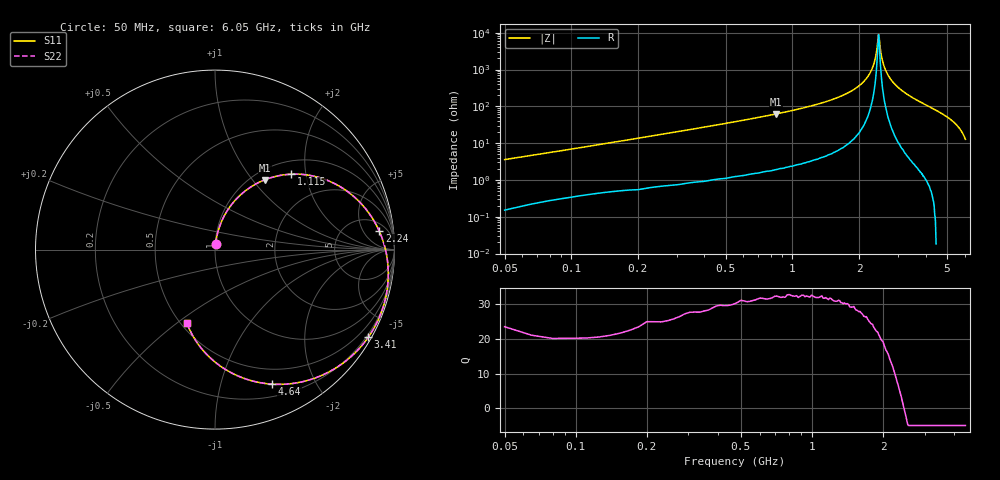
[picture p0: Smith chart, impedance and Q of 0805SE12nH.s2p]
! AVX Thin Film Operation		Date: May 2002
! Description: Accu-L® Series, Thin Film, SMD, RF Inductors
! Part Number: L0805120GEWTR
! 50 MHz  -  6.05 GHz
! Serial Measurements
# mhz S db R 50
!	S11		S21		S12		S22
!	dB	Phase	dB	Phase	dB	Phase	dB	Phase
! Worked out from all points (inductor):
!   401 points, 50 MHz to 6.05 GHz, reference 50 ohm
!   read as 1/Y11, port 2 shorted: L = 10.9 nH near 80 MHz
!   highest Q = 32.5 at 845 MHz (marker M1), where L = 11.7 nH
!   self-resonance near 2.45 GHz
!   S11 on the Smith chart (normalised r, x): 50 MHz: 1.00, +0.07; 1.115 GHz: 1.27, +1.66; 2.24 GHz: 9, +12; 3.41 GHz: 0.12, -3.76; 4.64 GHz: 0.33, -1.46; 6.05 GHz: 0.54, -0.54
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50  -29.56 84.5  -0.01 -2.2  -0.01 -2.2  -29.56 84.5
155  -20.28 80.8  -0.08 -6.4  -0.08 -6.4  -20.28 80.8
305  -14.60 75.2  -0.21 -12.4  -0.21 -12.4  -14.60 75.2
530  -10.07 66.6  -0.54 -21.2  -0.54 -21.2  -10.07 66.6
845  -6.44 54.6  -1.24 -33.1  -1.24 -33.1  -6.44 54.6
1055  -4.84 46.8  -1.88 -40.8  -1.88 -40.8  -4.84 46.8
1115  -4.46 44.6  -2.08 -42.9  -2.09 -42.9  -4.46 44.6
1550  -2.41 29.2  -3.96 -57.9  -3.96 -57.9  -2.41 29.2
2060  -1.03 12.2  -7.26 -74.1  -7.26 -74.1  -1.03 12.2
2240  -0.71 6.4  -8.87 -79.5  -8.87 -79.5  -0.71 6.4
2795  -0.16 -11.0  -17.60 -93.8  -17.60 -93.8  -0.16 -11.0
2960  -0.10 -16.1  -23.82 -93.8  -23.80 -93.8  -0.10 -16.1
3050  -0.09 -18.8  -30.56 -72.8  -30.60 -72.8  -0.09 -18.8
3095  -0.08 -20.2  -37.64 -54.6  -37.60 -54.6  -0.08 -20.2
3125  -0.08 -21.1  -35.31 -25.6  -35.30 -25.6  -0.08 -21.1
3260  -0.10 -25.2  -24.57 58.5  -24.60 58.5  -0.10 -25.2
3410  -0.14 -29.8  -18.51 59.8  -18.50 59.8  -0.14 -29.8
3680  -0.31 -38.0  -12.98 54.1  -13.00 54.1  -0.31 -38.0
4055  -0.72 -49.3  -8.75 44.3  -8.75 44.3  -0.72 -49.3
4640  -1.79 -67.1  -4.99 28.2  -4.99 28.2  -1.79 -67.1
5060  -2.93 -79.9  -3.30 16.7  -3.30 16.7  -2.93 -79.9
6050  -7.17 -111.0  -1.08 -9.1  -1.08 -9.1  -7.17 -111.0
